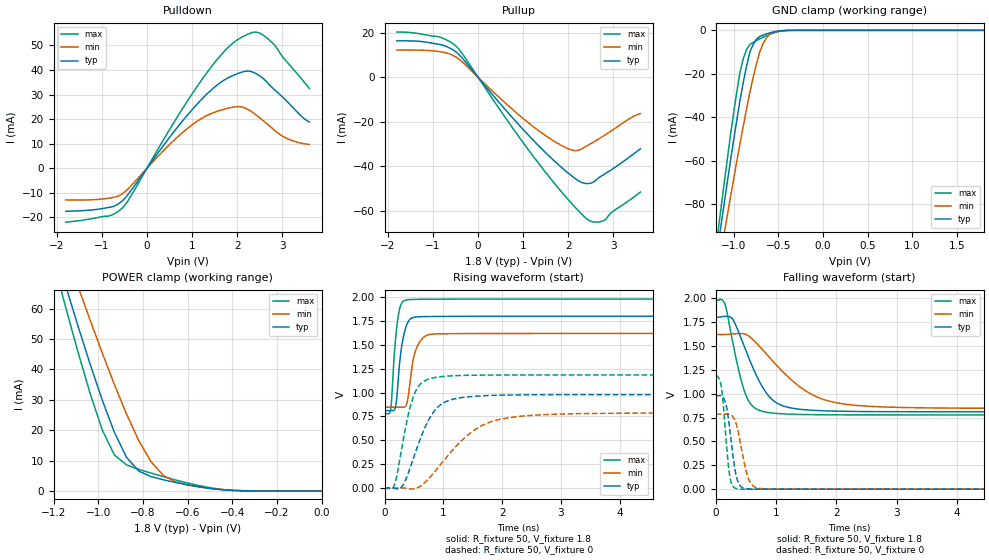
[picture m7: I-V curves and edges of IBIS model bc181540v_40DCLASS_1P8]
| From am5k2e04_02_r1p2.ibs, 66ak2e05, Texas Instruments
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|   Model Cell bc181540v_40DCLASS_1P8
|bc181540v_40DCLASS_1P8
[Model]   bc181540v_40DCLASS_1P8
Model_type   I/O
Polarity   Non-Inverting
Enable   Active-Low
Vinl =  0.63
Vinh =  1.17
Cref =  15.0000pF
Rref =  100.0000M
Vref =  0V
Vmeas =  0.9
C_comp   1.16613p   0.553312p   1.16742p
[Model Spec]
Vinl   0.63   0.567   0.693
Vinh   1.17   1.053   1.287
[Temperature Range]   25   125   -40
[Voltage Range]   1.8   1.62   1.98
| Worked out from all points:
|   slope of the pulldown table from 0 to 0.27 V, typ, clamps not added: 39.2 ohm
|   slope of the pullup table from 0 to 0.27 V, typ, clamps not added: 40.9 ohm
|   GND clamp passes 1 mA (typ) near -0.58 V on its own axis
|   POWER clamp passes 1 mA (typ) near -0.52 V on its own axis
|   rising waveform, R_fixture 50, V_fixture 1.8: 20-80 % time 110ps typ, 131ps min, 89.1ps max; typ from 0.811 V to 1.8 V
|   rising waveform, R_fixture 50, V_fixture 0: 20-80 % time 392ps typ, 749ps min, 243ps max; typ from 0 V to 0.979 V
|   falling waveform, R_fixture 50, V_fixture 1.8: 20-80 % time 431ps typ, 797ps min, 260ps max; typ from 1.8 V to 0.811 V
|   falling waveform, R_fixture 50, V_fixture 0: 20-80 % time 121ps typ, 155ps min, 95.7ps max; typ from 0.979 V to 0 V
[POWER_clamp]
|   voltage   I(typ)   I(min)   I(max)
-1.8V     235.9mA    223mA      250.7mA
-1.164V   71.87mA    82.65mA    65.36mA
-1.127V   63.07mA    75mA       55.51mA
-1.073V   50.17mA    63.68mA    41.25mA
-981.8mV  29.88mA    45.37mA    20.07mA
-927.3mV  19.23mA    34.95mA    11.8mA
-872.7mV  11mA       25.21mA    8.54mA
-818.2mV  6.508mA    16.53mA    7.086mA
-763.6mV  4.722mA    9.611mA    5.869mA
-709.1mV  3.682mA    5.172mA    4.713mA
-490.9mV  715.9uA    765.4uA    948.8uA
0V        973.6pA    18.39nA    2.408nA
[Pulldown]
|   voltage   I(typ)   I(min)   I(max)
-1.8V     -17.49mA   -12.88mA   -21.94mA
-818.2mV  -15.86mA   -12.08mA   -19.3mA
-545.5mV  -13.25mA   -10.42mA   -16.15mA
490.9mV   12.32mA    9.498mA    15.44mA
1.036V    24.59mA    18.17mA    31.25mA
1.691V    35.67mA    23.94mA    47.16mA
2.127V    39.29mA    24.81mA    53.62mA
2.4V      38.7mA     21.96mA    55.46mA
2.618V    35.92mA    18.78mA    53.67mA
2.836V    31.87mA    15.36mA    50.01mA
3.055V    28.14mA    12.57mA    44.34mA
3.6V      18.85mA    9.7mA      32.48mA
[Pullup]
|   voltage   I(typ)   I(min)   I(max)
-1.8V     16.38mA    12.23mA    20.34mA
-872.7mV  14.84mA    11.61mA    18.24mA
-490.9mV  11.44mA    9.116mA    14.06mA
818.2mV   -19.46mA   -15.43mA   -24.31mA
1.582V    -35.6mA    -27.44mA   -44.98mA
2.127V    -45.2mA    -32.99mA   -57.98mA
2.291V    -47.33mA   -32.3mA    -61.49mA
2.455V    -47.84mA   -30.39mA   -64.41mA
2.618V    -46.24mA   -28.46mA   -65.26mA
2.782V    -43.87mA   -26.41mA   -64.63mA
2.945V    -41.78mA   -24.25mA   -61.08mA
3.6V      -32.22mA   -16.39mA   -51.67mA
[GND_clamp]
|   voltage   I(typ)   I(min)   I(max)
-1.8V     -286.5mA   -268.3mA   -306.4mA
-1.182V   -101.5mA   -112.2mA   -95.12mA
-1.145V   -91mA      -103.2mA   -83.18mA
-1.109V   -80.68mA   -94.46mA   -71.51mA
-1.073V   -70.47mA   -85.72mA   -60.02mA
-927.3mV  -31.93mA   -51.83mA   -19.01mA
-890.9mV  -23.7mA    -43.85mA   -12.93mA
-818.2mV  -10.01mA   -28.59mA   -6.521mA
-709.1mV  -2.875mA   -10.12mA   -3.938mA
-600mV    -1.201mA   -1.844mA   -1.918mA
-490.9mV  -279uA     -308.3uA   -510uA
1.8V      973.6pA    1.906uA    493.4pA
[Ramp]
| variable   typ   min   max
dV/dt_f   0.599958/0.43371488n   0.470178/0.80244779n   0.728094/0.26114761n
dV/dt_r   0.594354/0.39533169n  0.4784664/0.75562064n 0.71589888/0.2435884n
R_load = 50
[Rising Waveform]
R_fixture = 50
V_fixture = 1.8
V_fixture_min = 1.62
V_fixture_max = 1.98
|   time   V(typ)   V(min)   V(max)
0s        810.7mV    846.4mV    777.9mV
104.3ps   810.8mV    846.4mV    827.7mV
181.7ps   840.4mV    846.3mV    1.536V
262.7ps   1.357V     846.4mV    1.896V
320.7ps   1.588V     845.9mV    1.959V
393.7ps   1.735V     931mV      1.973V
467.7ps   1.782V     1.283V     1.976V
536.1ps   1.792V     1.456V     1.977V
830.2ps   1.798V     1.613V     1.979V
16.75ns   1.8V       1.62V      1.98V
[Rising Waveform]
R_fixture = 50
V_fixture = 0
V_fixture_min = 0
V_fixture_max = 0
|   time   V(typ)   V(min)   V(max)
0s        0V         0V         0V
177.9ps   -5.336mV   0V         53.9mV
319.3ps   37.18mV    0V         513.5mV
433.6ps   210.7mV    -9.243mV   848mV
533.7ps   390.6mV    0V         1.024V
733.5ps   695.6mV    86.73mV    1.138V
945.3ps   869.8mV    241mV      1.166V
1.633ns   965.5mV    646.9mV    1.183V
2.586ns   977.4mV    764.8mV    1.185V
16.71ns   978.8mV    786.4mV    1.185V
[Falling Waveform]
R_fixture = 50
V_fixture = 1.8
V_fixture_min = 1.62
V_fixture_max = 1.98
|   time   V(typ)   V(min)   V(max)
0s        1.801V     1.62V      1.98V
162.3ps   1.81V      1.62V      1.921V
290.2ps   1.772V     1.627V     1.512V
424.4ps   1.575V     1.63V      1.136V
537.6ps   1.392V     1.609V     933.1mV
739.4ps   1.11V      1.487V     822.3mV
914.8ps   951.9mV    1.363V     798.8mV
1.617ns   825.8mV    984.7mV    780.3mV
2.527ns   812.8mV    868.4mV    778.1mV
16.75ns   810.7mV    846.4mV    777.9mV
[Falling Waveform]
R_fixture = 50
V_fixture = 0
V_fixture_min = 0
V_fixture_max = 0
|   time   V(typ)   V(min)   V(max)
0s        978.8mV    786.4mV    1.185V
95.5ps    976.9mV    786.4mV    1.061V
179.7ps   862.9mV    786.3mV    457mV
244.6ps   563.5mV    782.6mV    96.11mV
328.7ps   172.4mV    703.1mV    8.681mV
404.3ps   36.05mV    499.7mV    0V
498.4ps   5.701mV    202.6mV    0V
567.7ps   2.229mV    76.03mV    0V
864.1ps   0V         0V         0V
16.71ns   0V         0V         0V
